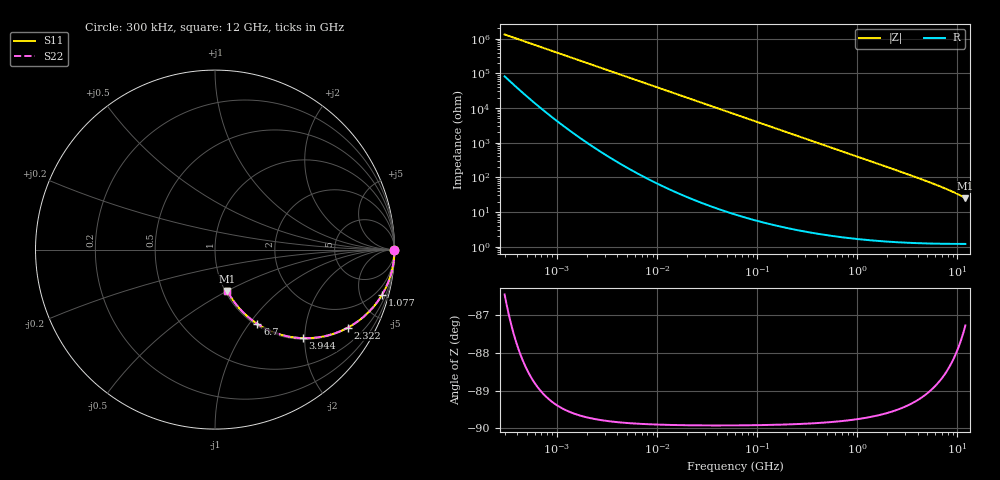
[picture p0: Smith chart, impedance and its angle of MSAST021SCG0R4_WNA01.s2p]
! MSAST021SCG0R4_WNA01  S-PARAMETER MODEL  ( General Type )
! Model Generated by TAIYO YUDEN Corporation (http://www.ty-top.com)
! Version 2.0
! TAIYO YUDEN Control No. 181101
! Copyright(c) 2015 TAIYO YUDEN CO.,LTD. All Rights Reserved.
! Product Description (link to TY-COMPAS)
! https://ds.yuden.co.jp/TYCOMPAS/or/detail?pn=MSAST021SCG0R4BWNA01&u=M
! Products Name : Multilayer Ceramic Capacitors
! Characteristics :
!  Capacitance : 0.4 pF , Rated Voltage : 25V , TCC : CG / C0G
!  Case Size : 0.25 x 0.125 / 0.0098 x 0.0049 [mm/inch] , Thickness : 0.125 / 0.0049 [mm/inch]
!  (Conditions: Temperature = 25 degC , DC Bias Current/Voltage = 0A / 0V)
! External Node Assignments :
!  1  o---| |---o  2
! GND o---------o GND
! Frequency Range : 0.3MHz  -  12000MHz  [ 401 STEP ]
# MHz S RI R 50
! Freq[MHz].  S11 Real  S11 Imag  S21 Real  S21 Imag  S12 Real  S12 Imag  S22 Real  S22 Imag
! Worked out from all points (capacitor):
!   401 points, 300 kHz to 12 GHz, reference 50 ohm
!   read as one part in series: C = 400 fF near 316.3 kHz
!   lowest |Z| = 25.1 ohm at 12 GHz (marker M1)
!   S11 on the Smith chart (normalised r, x): 300 kHz: open; 1.077 GHz: 1.03, -7.37; 2.322 GHz: 1.03, -3.39; 3.944 GHz: 1.03, -1.96; 6.7 GHz: 1.02, -1.10; 12 GHz: 1.02, -0.50
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0.3  1 -7.52e-05  4.67e-06 7.52e-05  4.67e-06 7.52e-05  1 -7.52e-05
0.380774  1 -9.56e-05  4e-06 9.56e-05  4e-06 9.56e-05  1 -9.56e-05
0.412271  1 -0.000104  3.82e-06 0.000104  3.82e-06 0.000104  1 -0.000104
1.769972  1 -0.000445  2.7e-06 0.000445  2.7e-06 0.000445  1 -0.000445
10.44266  1 -0.00263  1.12e-05 0.00263  1.12e-05 0.00263  1 -0.00263
60  0.9998 -0.0151  0.000247 0.0151  0.000247 0.0151  0.9998 -0.0151
164.1901  0.9982 -0.0412  0.00177 0.0412  0.00177 0.0412  0.9982 -0.0412
353.9943  0.9919 -0.0883  0.00807 0.0883  0.00807 0.0883  0.9919 -0.0883
634.0297  0.9747 -0.1555  0.0253 0.1555  0.0253 0.1555  0.9747 -0.1555
848.5281  0.9556 -0.2041  0.0444 0.2041  0.0444 0.2041  0.9556 -0.2041
1076.992  0.9304 -0.2523  0.0696 0.2523  0.0696 0.2523  0.9304 -0.2523
1519.776  0.8702 -0.3333  0.1298 0.3333  0.1298 0.3333  0.8702 -0.3333
2088.533  0.7794 -0.411  0.2206 0.411  0.2206 0.411  0.7794 -0.411
2321.999  0.7404 -0.4344  0.2596 0.4344  0.2596 0.4344  0.7404 -0.4344
3107.553  0.6117 -0.4822  0.3883 0.4822  0.3883 0.4822  0.6117 -0.4822
3944.255  0.4907 -0.4935  0.5093 0.4935  0.5093 0.4935  0.4907 -0.4935
5140.631  0.3554 -0.4704  0.6446 0.4704  0.6446 0.4704  0.3554 -0.4704
6699.894  0.2361 -0.4138  0.7639 0.4138  0.7639 0.4138  0.2361 -0.4138
8966.534  0.1357 -0.3271  0.8643 0.3271  0.8643 0.3271  0.1357 -0.3271
10511.28  0.0954 -0.2749  0.9046 0.2749  0.9046 0.2749  0.0954 -0.2749
11380.75  0.0788 -0.2484  0.9212 0.2484  0.9212 0.2484  0.0788 -0.2484
12000  0.0689 -0.2306  0.9311 0.2306  0.9311 0.2306  0.0689 -0.2306
